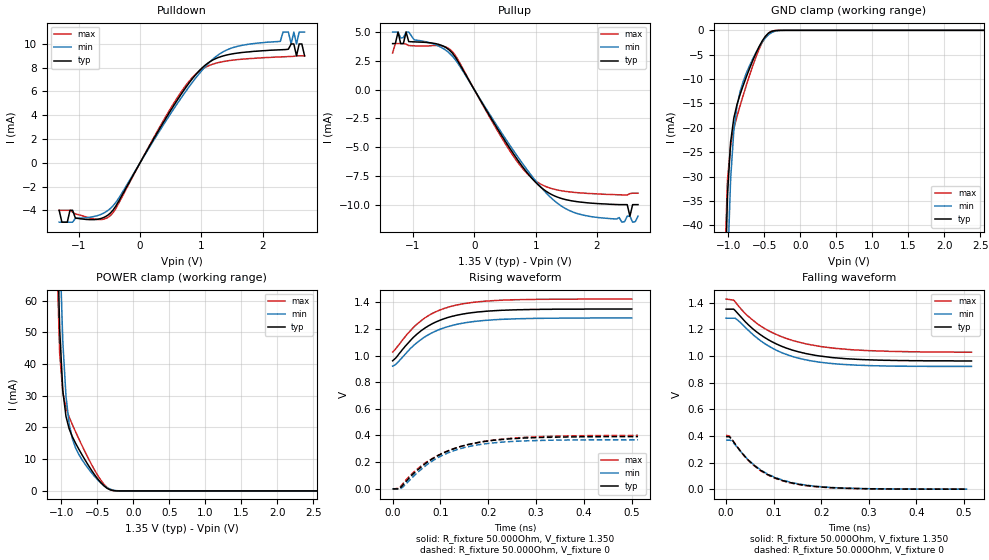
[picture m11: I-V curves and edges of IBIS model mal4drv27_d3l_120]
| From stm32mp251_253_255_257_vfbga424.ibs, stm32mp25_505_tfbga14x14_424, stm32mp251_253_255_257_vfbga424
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[Model] mal4drv27_d3l_120
Model_type   I/O
Polarity   Non-Inverting
Enable   Active-High
C_comp   1.684pF   1.663pF   1.711pF
C_comp_pullup   812.334fF   800.254fF   826.800fF
C_comp_pulldown   769.309fF   756.111fF   787.425fF
Vinh = 805.000mV
Vinl = 545.000mV
Vmeas = 675.000mV
Vref = 675.000mV
Rref = 50Ohms
Cref = 0pF
[Model Spec]
Vinh   805.000mV   772.000mV   855.000mV
Vinl   545.000mV   512.000mV   595.000mV
Vmeas   675.000mV   642.000mV   725.000mV
Vref   675.000mV   642.000mV   725.000mV
D_overshoot_ampl_h 0.4 NA   NA
D_overshoot_ampl_l 0.4 NA   NA
D_overshoot_area_l 110.000m NA   NA
D_overshoot_area_h 110.000m NA   NA
[Temperature Range]   25.000   125.000   -40.000
[Voltage Range]   1.350V   1.283V   1.425V
[GND Clamp Reference]   0.00V   0.00V   0.00V
[C Comp Corner]
| variable   typ   min   max
C_comp   1.684pF   1.663pF   1.711pF
C_comp_pullup   812.334fF   800.254fF   826.800fF
C_comp_pulldown   769.309fF   756.111fF   787.425fF
[Pulldown Reference]   0.00V   0.00V   0.00V
[POWER Clamp Reference]   1.350V   1.283V   1.425V
[Pullup Reference]   1.350V   1.283V   1.425V
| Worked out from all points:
|   slope of the pulldown table from 0 to 0.203 V, typ, clamps not added: 110 ohm
|   slope of the pullup table from 0 to 0.203 V, typ, clamps not added: 110 ohm
|   GND clamp passes 1 mA (typ) near -0.47 V on its own axis
|   POWER clamp passes 1 mA (typ) near -0.37 V on its own axis
|   rising waveform, R_fixture 50.000Ohm, V_fixture 1.350: 20-80 % time 84.4ps typ, 87.2ps min, 82.3ps max; typ from 0.961 V to 1.35 V
|   rising waveform, R_fixture 50.000Ohm, V_fixture 0: 20-80 % time 104ps typ, 96.5ps min, 115ps max; typ from -0.001 V to 0.391 V
|   falling waveform, R_fixture 50.000Ohm, V_fixture 1.350: 20-80 % time 107ps typ, 100ps min, 116ps max; typ from 1.35 V to 0.963 V
|   falling waveform, R_fixture 50.000Ohm, V_fixture 0: 20-80 % time 83.3ps typ, 86.4ps min, 81.6ps max; typ from 0.394 V to 0 V
[GND Clamp]
-1.318V   -672mA     -638mA     -661.1mA
-1.054V   -60.41mA   -84.99mA   -50.75mA
-1.011V   -34.02mA   -49.92mA   -30.84mA
-966.7mV  -22.91mA   -30.54mA   -23.58mA
-922.7mV  -18.04mA   -20.68mA   -20.16mA
-878.8mV  -15.25mA   -15.56mA   -17.69mA
-834.8mV  -13.14mA   -12.55mA   -15.44mA
-747mV    -9.486mA   -8.743mA   -11.21mA
-615.2mV  -4.709mA   -4.591mA   -5.504mA
-439.4mV  -562.2uA   -889.5uA   -546.1uA
-219.7mV  -954.1nA   -9.356uA   -215nA
2.68V     18.98nA    945nA      23.53nA
[Power Clamp]
-1.33V    889mA      842.2mA    872.8mA
-1.067V   94.44mA    130.9mA    77.96mA
-1.023V   51.04mA    78.45mA    43.53mA
-978.8mV  31.54mA    46.94mA    31.01mA
-934.8mV  23.45mA    29.85mA    26.15mA
-890.9mV  19.58mA    21.13mA    23.3mA
-847mV    17.11mA    16.47mA    20.93mA
-671.2mV  9.815mA    8.474mA    12.37mA
-495.5mV  3.823mA    3.529mA    4.955mA
-363.6mV  819.5uA    1.024mA    1.072mA
-187.9mV  4.227uA    28.6uA     2.566uA
2.668V    -29.12nA   -796.8nA   -15.73nA
[Pulldown]
-1.318V   -4mA       -5mA       -4mA
-1.274V   -5mA       -5mA       -4mA
-1.142V   -4mA       -5mA       -4mA
-483.3mV  -4.228mA   -3.844mA   -4.446mA
615.2mV   5.344mA    5.046mA    5.544mA
1.142V    8.521mA    8.516mA    8.221mA
2.329V    9.52mA     11mA       8.919mA
2.461V    10mA       10mA       8.95mA
2.505V    10mA       11mA       8.96mA
2.549V    9mA        10mA       9mA
2.592V    10mA       11mA       9mA
2.68V     9mA        11mA       9mA
[Pullup]
-1.33V    4mA        5mA        3.193mA
-1.242V   5mA        5mA        4mA
-1.155V   4mA        4.526mA    4mA
-1.111V   5mA        5mA        3.952mA
-1.067V   4.17mA     5mA        3.827mA
-407.6mV  3.441mA    3.181mA    3.543mA
734.8mV   -6.32mA    -6.036mA   -6.506mA
1.35V     -9.334mA   -9.855mA   -8.72mA
2.492V    -10mA      -11mA      -9.16mA
2.536V    -11mA      -11mA      -9.042mA
2.58V     -10mA      -11.53mA   -9mA
2.668V    -10mA      -11mA      -9mA
[Ramp]
R_load=50.000Ohm
dV/dt_r   233.700mV/95.000ps  218.998mV/93.000ps  239.400mV/99.500ps
dV/dt_f   233.700mV/96.000ps  218.998mV/95.000ps  239.400mV/100.000ps
[Rising waveform]
R_fixture=50.000Ohm
V_fixture=1.350
V_fixture_min=1.283
V_fixture_max=1.425
0s        961mV      921mV      1.027V
10ps      997mV      946mV      1.068V
39ps      1.121V     1.06V      1.196V
62ps      1.193V     1.128V     1.27V
91ps      1.254V     1.186V     1.331V
133ps     1.303V     1.234V     1.38V
177ps     1.328V     1.259V     1.403V
234ps     1.341V     1.274V     1.417V
334ps     1.349V     1.281V     1.424V
500ps     1.35V      1.283V     1.425V
[Rising waveform]
R_fixture=50.000Ohm
V_fixture=0
0s        -1.476mV   -1.805mV   -3.755mV
14ps      -1.476mV   -1.805mV   4.533mV
17ps      8.986mV    621uV      17.8mV
45ps      118mV      98.15mV    128mV
79ps      215mV      199mV      219mV
121ps     291mV      277mV      291mV
169ps     341mV      324mV      340mV
213ps     364mV      345mV      367mV
285ps     382mV      360mV      388mV
513ps     391mV      367mV      401mV
[Falling waveform]
R_fixture=50.000Ohm
V_fixture=1.350
V_fixture_min=1.283
V_fixture_max=1.425
0s        1.352V     1.284V     1.428V
16ps      1.352V     1.284V     1.42V
19ps      1.342V     1.284V     1.408V
47ps      1.234V     1.192V     1.296V
79ps      1.144V     1.099V     1.211V
122ps     1.066V     1.018V     1.138V
168ps     1.018V     971mV      1.092V
221ps     989mV      944mV      1.062V
300ps     972mV      928mV      1.04V
516ps     963mV      922mV      1.029V
[Falling waveform]
R_fixture=50.000Ohm
V_fixture=0
0s        394mV      368mV      404mV
7ps       394mV      368mV      400mV
14ps      364mV      354mV      365mV
45ps      225mV      227mV      222mV
71ps      146mV      149mV      142mV
100ps     89.17mV    93.2mV     86.27mV
139ps     45.99mV    49.26mV    43.55mV
180ps     23.14mV    25.04mV    21.49mV
242ps     7.943mV    8.984mV    7.03mV
507ps     74.86uV    115.7uV    61.56uV
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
